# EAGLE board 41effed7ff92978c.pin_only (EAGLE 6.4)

Size 20.32 x 60.96 mm. Coordinates in mm from the lower left corner, seen from the top.
Outline: 19.05,60.96 1.27,60.96 arc90 0,59.69 0,1.27 arc90 1.27,0 19.05,0 arc90 20.32,1.27 20.32,59.69 arc90 19.05,60.96
Copper layers (1*16): Top 0.035mm / dielectric 1.5mm / Bottom 0.035mm
Design rules "adafruit": minimum track width 8mil, minimum drill 15.5mil, track to track 8mil, track to pad 8mil, pad to pad 8mil, via to via 8mil, smd to smd 8mil, copper to edge 10mil, drill to drill 8mil, minimum pad ring 10mil, minimum via ring 8mil, stop-mask expansion 4mil, vias tented up to drill 20mil, thermal gap 10mil

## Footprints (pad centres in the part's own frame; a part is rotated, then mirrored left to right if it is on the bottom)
PADS-14 = drill 1.016 pad 1.778: 1 -16.51,0; 2 -13.97,0; 3 -11.43,0; 4 -8.89,0; 5 -6.35,0; 6 -3.81,0; 7 -1.27,0; 8 1.27,0; 9 3.81,0; 10 6.35,0; 11 8.89,0; 12 11.43,0; 13 13.97,0; 14 16.51,0
PADS-10 = drill 1.016 pad 1.778: 1 -11.43,0; 2 -8.89,0; 3 -6.35,0; 4 -3.81,0; 5 -1.27,0; 6 1.27,0; 7 3.81,0; 8 6.35,0; 9 8.89,0; 10 11.43,0
BREAKOUTS_TQFP48 = smd 1.5 x 0.275: 1 -4.3,2.75; 2 -4.3,2.25; 3 -4.3,1.75; 4 -4.3,1.25; 5 -4.3,0.75; 6 -4.3,0.25; 7 -4.3,-0.25; 8 -4.3,-0.75; 9 -4.3,-1.25; 10 -4.3,-1.75; 11 -4.3,-2.25; 12 -4.3,-2.75; 25 4.3,-2.75; 26 4.3,-2.25; 27 4.3,-1.75; 28 4.3,-1.25; 29 4.3,-0.75; 30 4.3,-0.25; 31 4.3,0.25; 32 4.3,0.75; 33 4.3,1.25; 34 4.3,1.75; 35 4.3,2.25; 36 4.3,2.75 | smd 0.275 x 1.5: 13 -2.75,-4.3; 14 -2.25,-4.3; 15 -1.75,-4.3; 16 -1.25,-4.3; 17 -0.75,-4.3; 18 -0.25,-4.3; 19 0.25,-4.3; 20 0.75,-4.3; 21 1.25,-4.3; 22 1.75,-4.3; 23 2.25,-4.3; 24 2.75,-4.3; 37 2.75,4.3; 38 2.25,4.3; 39 1.75,4.3; 40 1.25,4.3; 41 0.75,4.3; 42 0.25,4.3; 43 -0.25,4.3; 44 -0.75,4.3; 45 -1.25,4.3; 46 -1.75,4.3; 47 -2.25,4.3; 48 -2.75,4.3
BREAKOUTS_QFN48 = smd 0.9 x 0.275: 1 -3.475,2.75; 12 -3.475,-2.75; 25 3.475,-2.75; 36 3.475,2.75 | smd 0.95 x 0.275: 2 -3.475,2.25; 3 -3.475,1.75; 4 -3.475,1.25; 5 -3.475,0.75; 6 -3.475,0.25; 7 -3.475,-0.25; 8 -3.475,-0.75; 9 -3.475,-1.25; 10 -3.475,-1.75; 11 -3.475,-2.25; 26 3.475,-2.25; 27 3.475,-1.75; 28 3.475,-1.25; 29 3.475,-0.75; 30 3.475,-0.25; 31 3.475,0.25; 32 3.475,0.75; 33 3.475,1.25; 34 3.475,1.75; 35 3.475,2.25 | smd 0.275 x 0.9: 13 -2.75,-3.475; 24 2.75,-3.475; 37 2.75,3.475; 48 -2.75,3.475 | smd 0.275 x 0.95: 14 -2.25,-3.475; 15 -1.75,-3.475; 16 -1.25,-3.475; 17 -0.75,-3.475; 18 -0.25,-3.475; 19 0.25,-3.475; 20 0.75,-3.475; 21 1.25,-3.475; 22 1.75,-3.475; 23 2.25,-3.475; 38 2.25,3.475; 39 1.75,3.475; 40 1.25,3.475; 41 0.75,3.475; 42 0.25,3.475; 43 -0.25,3.475; 44 -0.75,3.475; 45 -1.25,3.475; 46 -1.75,3.475; 47 -2.25,3.475 | smd 5.309 x 5.309: EXP 0,0

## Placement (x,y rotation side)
JP1  [PADS-14]  1.27,43.18 270 top
JP2  [PADS-14]  19.05,43.18 270 top
JP3  [PADS-10]  1.27,12.7 270 top
JP4  [PADS-10]  19.05,12.7 270 top
U$1  BREAKOUTS_48-PINTQFP  [BREAKOUTS_TQFP48]  10.16,30.48 315 top
U$2  BREAKOUTS_48-PINQFN  [BREAKOUTS_QFN48]  10.16,30.48 315 bottom
U$3  [ADAFRUIT_3.5MM]  8.26,55.88 0 top
U$4  [ADAFRUIT_3.5MM]  12.06,55.88 0 bottom

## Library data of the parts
JP1-JP4 = breakouts
U$1 U$2 = fpp48-pin
U$3 U$4 = microbuilder

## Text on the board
tPlace: 48 | 2 | 47 | 3 | 46 | 4 | 45 | 5 | 44 | 6 | 43 | 7 | 42 | 8 | 41 | 9 | 40 | 10 | 39 | 11 | 38 | 12 | 37 | 13 | 36 | 14 | 35 | 15 | 34 | 16 | 33 | 17 | 32 | 18 | 31 | 19 | 30 | 20 | 29 | 21 | 28 | 22 | 27 | 23 | 7x7mm | 26 | TQFP-48 | 24 | 25
bPlace: 48 | 47 | 2 | 46 | 3 | 45 | 4 | 44 | 5 | 43 | 6 | 42 | 7 | 41 | 8 | 40 | 9 | 39 | 10 | 38 | 11 | 37 | 12 | 36 | 13 | 35 | 14 | 34 | 15 | 33 | 16 | 32 | 17 | 31 | 18 | 30 | 19 | 29 | 20 | 28 | 21 | 27 | 22 | 26 | 7x7mm | 23 | QFN-48 | 25 | 24

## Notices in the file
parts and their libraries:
microbuilder: This work is placed in the public domain, and may be freely used for commercial and non-commercial work with the following conditions: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
